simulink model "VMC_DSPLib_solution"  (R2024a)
settings: Solver=VariableStepDiscrete  StartTime=0.0  StopTime=5000  RelTol=1e-3
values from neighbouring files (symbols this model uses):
  cfi = NormalizeCoef(cf.Numerator,Kcf)    [CreateFilter.m]
  hb1 = NormalizeHBCoef(hb.Numerator,K1/2)    [CreateFilter.m]
  hb2 = NormalizeHBCoef(hb.Numerator,K2/2)    [CreateFilter.m]
  hb3 = NormalizeHBCoef(hb.Numerator,K3/2)    [CreateFilter.m]
  S = sum(round(C0))    [NormalizeCoef.m]
  Shift2 = 15    [CreateFilter.m]
  Shift3 = 15    [CreateFilter.m]
  ShiftCF = 15    [CreateFilter.m]
undefined symbols (not defined in the file or in its folder): aiecode_src, code, Evaluation, FreqShift, None, Platform, VCK190, Versal, vsva2197, xcvc1902
libraries: aieDSP x4, aieBasic x3, dspmlti4 x3, dspsrcs4 x1, aieUtilities x1, vmcUtilities x1

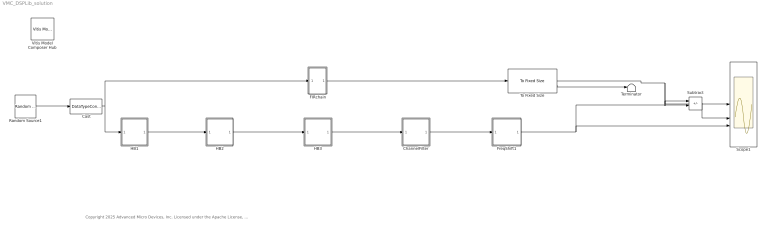
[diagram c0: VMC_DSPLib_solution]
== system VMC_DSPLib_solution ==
  note: Copyright 2025 Advanced Micro Devices, Inc. Licensed under the Apache License, Version 2.0 (the "License"); you may not use this file except in compliance with the License. You may obtain a copy of the License at http://www.apache.org/licenses/LICENSE-2.0 Unless required by applicable law or agreed to in writing, software distributed under the License is distributed on an "AS IS" BASIS, WITHOUT WARRANTIES OR CONDITIONS OF ANY KIND, either express or implied. See the License for the specific language governing permissions and limitations under the License.
  Cast : DataTypeConversion  OutDataTypeStr=int16
  ChannelFilter : Subsystem  mask{COEFFS=cfi, Shift=ShiftCF}
      mask prompts: COEFFS "Coefficients"; Shift "Final Shift"
  FIRchain : Subsystem
  FreqShift1 : Subsystem
  HB1 : Subsystem  mask{COEFFS=hb1, Shift=16}
      mask prompts: COEFFS "Coefficients"; Shift "Final Shift"
  HB2 : Subsystem  mask{COEFFS=hb2, Shift=Shift2}
      mask prompts: COEFFS "Coefficients"; Shift "Final Shift"
  HB3 : Subsystem  mask{COEFFS=hb3, Shift=Shift3}
      mask prompts: COEFFS "Coefficients"; Shift "Final Shift"
  Random Source1 : dspsrcs4/Random Source  SrcType=Uniform  MinVal=-30000  MaxVal=30000  MeanVal=0  VarVal=1  RepMode=Specify seed  rawSeed=1  IsInherit=off  SampTime=1  SampFrame=2048  OutComplex=Complex  DataType=double  SimulateUsing=Interpreted execution
  Scope1 : Scope  NumInputPorts=3
  Subtract : Sum  Inputs=+-
  Terminator : Terminator
  To Fixed Size : aieUtilities/To Fixed Size  Mode=Produce a valid output signal  OutputSize=256  CopyMethod=Buffer samples to form output  HasStatusOutput=on
  Vitis Model Composer Hub : vmcUtilities/Vitis Model Composer Hub  Tag=genX  CodeGeneration=off  SubsystemName=FIRchain  StartColumn=1  NumberOfColumns=1  TargetDirectory=./code  exportDesign=off  analyzeDesign=off  validateDesignOnHw=off  ExportType=AI Engines  IpVendor=xilinx.com  IpLibrary=hls  IpVersion=1.0  IpHWLanguage=Verilog  AieCompilerOptions={}  AieSimulatorOptions={}  CreateTestbench=on  TestbenchStackSize=10  RunRtlSim=off  RunCSim=off  RunAieSim=on  AieSimTimeout=50000  RunAieSimProfiling=on  LaunchVitisAnalyzer=on  PlotOutput=off  RunX86Sim=off  X86SimTimeout=10  GenHwImage=on  GenLibadfXo=off  GenHwValidationCode=off  PlatformType=Specify Platform  Platform=/opt/amd/Vitis/2024.2/base_platforms/xilinx_vck190_base_202420_1/xilinx_vck190_base_202420_1.xpfm  HwSystemType=Baremetal  HwValidationTarget=hw_emu  ProjDevice=Versal VCK190 Evaluation Platform (xcvc1902-vsva2197-2MP-e-S)  ProjDevicePart=xcvc1902-vsva2197-2MP-e-S  AIEType=AIE  SamplePeriod=-1  ClockFrequency=200  DataPathParallelism=1  xilinxfamily=versalaicore  part=xcvc1902  speed=-2MP-e-S  package=vsva2197  directory=./code  testbench=off  incr_netlist=off  synthesis_tool=Vivado  clock_wrapper=Clock Enables  dbl_ovrd=According to Block Masks  dcm_input_clock_period=10  sysclk_period=10  simulink_period=1  eval_field=0  IPInfoJsonString="{\"AIESubsystem\":{\"SubsystemName\":\"FIRchain\",\"TargetDirectory\":\"./code\",\"SubsystemDir\":\"./code/ip/FIRchain\"}}"  LogFileName=/home/amd/training/vmc_aie_dsplib/lab/VCK190/code/model_composer.log  NThreads=4
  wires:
  To Fixed Size/1 -> Subtract/1, Scope1/1
  Subtract/1 -> Scope1/2
  To Fixed Size/2 -> Terminator/1
  Cast/1 -> FIRchain/1(In1), HB1/1(In1)
  HB1/1(Out1) -> HB2/1(In1)
  HB2/1(Out1) -> HB3/1(In1)
  HB3/1(Out1) -> ChannelFilter/1(In1)
  ChannelFilter/1(Out1) -> FreqShift1/1(In1)
  FreqShift1/1(Out1) -> Subtract/2, Scope1/3
  FIRchain/1(Out1) -> To Fixed Size/1
  Random Source1/1 -> Cast/1

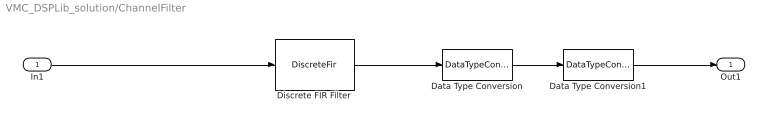
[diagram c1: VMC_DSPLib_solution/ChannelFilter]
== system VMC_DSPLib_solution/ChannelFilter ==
  In1 : Inport
  Data Type Conversion : DataTypeConversion  OutDataTypeStr=fixdt(1,32,Shift)  ConvertRealWorld=Stored Integer (SI)
  Data Type Conversion1 : DataTypeConversion  OutDataTypeStr=int16
  Discrete FIR Filter : DiscreteFir  Coefficients=COEFFS  InputProcessing=Columns as channels (frame based)
  Out1 : Outport
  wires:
  Data Type Conversion/1 -> Data Type Conversion1/1
  In1/1 -> Discrete FIR Filter/1
  Discrete FIR Filter/1 -> Data Type Conversion/1
  Data Type Conversion1/1 -> Out1/1

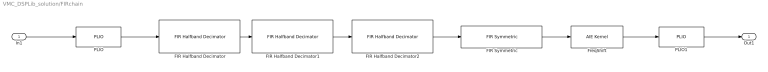
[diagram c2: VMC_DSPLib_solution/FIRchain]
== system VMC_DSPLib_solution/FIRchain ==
  In1 : Inport
  FIR Halfband Decimator : aieDSP/FIR Halfband Decimator  data_type=cint16  coef_type=int16  use_coeff_reload=off  dual_ip=off  num_outputs=off  coeff=hb1_aie  fir_length=31  input_window_size=2048  shift_val=16  rnd_mode=Floor  sat_mode=0-None  deci_poly=1  casc_length=2  AIE_VARIANT=1  blockJsonConstraints=[]  blockJsonConstraintsInternal=[]  spec=vmc_fir_decimate_hb.json  SerializedMaskParamNames=[]  SerializedMaskParamValues=[]  SerializedMaskParamVisibilities=[]  block_type=FIR Halfband Decimator  SerializedMaskParamDataypes=typename|typename|bool|bool|bool|coef_type|uint|uint|uint|uint|uint|uint|uint|uint  SerializedMaskParamEnumStrArr=0|0|0|0|0|0|0|0|0|Floor,Ceiling,Round to positive infinity,Round to negative infinity,Round symmetrical to infinity,Round symmetrical to zero,Round convergent to even,Round convergent to odd|0-None,1-Asymmetric,3-Symmetric|0|0|0  SerializedMaskParamEnumValArr=0|0|0|0|0|0|0|0|0|0,1,2,3,4,5,6,7|0,1,3|0|0|0  SerializedMaskParamVectorArr=0|0|0|0|0|1|0|0|0|0|0|0|0|0
  FIR Halfband Decimator1 : aieDSP/FIR Halfband Decimator  data_type=cint16  coef_type=int16  use_coeff_reload=off  dual_ip=off  num_outputs=off  coeff=hb2_aie  fir_length=31  input_window_size=1024  shift_val=Shift2  rnd_mode=Floor  sat_mode=0-None  deci_poly=1  casc_length=2  AIE_VARIANT=1  blockJsonConstraints=[]  blockJsonConstraintsInternal=[]  spec=vmc_fir_decimate_hb.json  SerializedMaskParamNames=[]  SerializedMaskParamValues=[]  SerializedMaskParamVisibilities=[]  block_type=FIR Halfband Decimator  SerializedMaskParamDataypes=typename|typename|bool|bool|bool|coef_type|uint|uint|uint|uint|uint|uint|uint|uint  SerializedMaskParamEnumStrArr=0|0|0|0|0|0|0|0|0|Floor,Ceiling,Round to positive infinity,Round to negative infinity,Round symmetrical to infinity,Round symmetrical to zero,Round convergent to even,Round convergent to odd|0-None,1-Asymmetric,3-Symmetric|0|0|0  SerializedMaskParamEnumValArr=0|0|0|0|0|0|0|0|0|0,1,2,3,4,5,6,7|0,1,3|0|0|0  SerializedMaskParamVectorArr=0|0|0|0|0|1|0|0|0|0|0|0|0|0
  FIR Halfband Decimator2 : aieDSP/FIR Halfband Decimator  data_type=cint16  coef_type=int16  use_coeff_reload=off  dual_ip=off  num_outputs=off  coeff=hb3_aie  fir_length=31  input_window_size=512  shift_val=Shift3  rnd_mode=Floor  sat_mode=0-None  deci_poly=1  casc_length=2  AIE_VARIANT=1  blockJsonConstraints=[]  blockJsonConstraintsInternal=[]  spec=vmc_fir_decimate_hb.json  SerializedMaskParamNames=[]  SerializedMaskParamValues=[]  SerializedMaskParamVisibilities=[]  block_type=FIR Halfband Decimator  SerializedMaskParamDataypes=typename|typename|bool|bool|bool|coef_type|uint|uint|uint|uint|uint|uint|uint|uint  SerializedMaskParamEnumStrArr=0|0|0|0|0|0|0|0|0|Floor,Ceiling,Round to positive infinity,Round to negative infinity,Round symmetrical to infinity,Round symmetrical to zero,Round convergent to even,Round convergent to odd|0-None,1-Asymmetric,3-Symmetric|0|0|0  SerializedMaskParamEnumValArr=0|0|0|0|0|0|0|0|0|0,1,2,3,4,5,6,7|0,1,3|0|0|0  SerializedMaskParamVectorArr=0|0|0|0|0|1|0|0|0|0|0|0|0|0
  FIR Symmetric : aieDSP/FIR Symmetric  data_type=cint16  coef_type=int16  use_coeff_reload=off  dual_ip=off  num_outputs=off  coeff=cfi_aie  fir_length=length(cfi)  input_window_size=256  shift_val=ShiftCF  rnd_mode=Floor  sat_mode=0-None  casc_length=1  AIE_VARIANT=1  blockJsonConstraints=[]  blockJsonConstraintsInternal=[]  spec=vmc_fir_sr_sym.json  SerializedMaskParamNames=[]  SerializedMaskParamValues=[]  SerializedMaskParamVisibilities=[]  block_type=FIR Symmetric  SerializedMaskParamDataypes=typename|typename|bool|bool|bool|coef_type|uint|uint|uint|uint|uint|uint|uint  SerializedMaskParamEnumStrArr=0|0|0|0|0|0|0|0|0|Floor,Ceiling,Round to positive infinity,Round to negative infinity,Round symmetrical to infinity,Round symmetrical to zero,Round convergent to even,Round convergent to odd|0-None,1-Asymmetric,3-Symmetric|0|0  SerializedMaskParamEnumValArr=0|0|0|0|0|0|0|0|0|0,1,2,3,4,5,6,7|0,1,3|0|0  SerializedMaskParamVectorArr=0|0|0|0|0|1|0|0|0|0|0|0|0
  FreqShift : aieBasic/AIE Kernel  KernelAllAttrs=s[12;12;9;9;19;14;21;23;21;23;24;21;15;17;12;24;26;26;26;27;28;9;21;23;23;23;24;25;14;19;19;29]@FunctionNameDeclFileNamePortNamesPortTypesPortSerializedTypesPortDirectionsPortWindowSizeEnablesPortWindowMarginEnablesPortBufferSizeEnablesPortBufferMarginEnablesPortSynchronicityEnablesPortSignalSizeEnablesPortBufferSizesPortBufferMarginsFunctionDeclFunctionTemplateSpecKindFunctionTemplateParamNamesFu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  PortNames={'in'; 'out'}  PortSerializedTypes={'{Q2{R{Tadf::input_buffer{1{t{Scint16}}}}}}'; '{Q2{R{Tadf::output_buffer{1{t{Scint16}}}}}}'}  PortWindowSizes={2.560000000000000000e+02, 2.560000000000000000e+02}  PortWindowMargins={0.000000000000000000e+00, 0.000000000000000000e+00}  PortSynchronicities={'sync', 'sync'}  PortSignalSizes={0.000000000000000000e+00; 0.000000000000000000e+00}  FunctionTemplateSpecKind=implicit  FunctionTemplateParamNames={'FRAME_LENGTH'}  FunctionTemplateParamKinds={'nontype'}  FunctionTemplateParamTypes={'int'}  FunctionTemplateParamValues={'256'}  FunctionIndex=1  FunctionTabVisible=on  FunctionTemplateParamsVisible=on  FunctionDeclTypeOptions=|  FunctionDecl=|  FunctionTemplateParams={ 'FRAME_LENGTH', 'int', '256' }  FunctionTemplateParamsEnables={'off', 'off', 'on'}  PortAttrs={ 'input', 'in', 'adf::input_buffer< cint16 > & restrict', '256', '0', 'sync', ''; 'output', 'out', 'adf::output_buffer< cint16 > & restrict', '256', '', 'sync', '' }  PortAttrsEnables={'off', 'off', 'off', 'on', 'off', 'off', 'off';'off', 'off', 'off', 'on', 'off', 'off', 'off'}  SampleTime=-1  KernelHeaderFile=aiecode_src/FreqShift.h  KernelFunction=FreqShift  KernelSourceFile=aiecode_src/FreqShift.cpp  KernelSearchPaths={}  PreProcOptions={}  blockJsonConstraints=[]
      | C[1 1]@t135@template < int FRAME_LENGTH > 
      | void FreqShift(adf::input_buffer< cint16 > && restrict in, adf::output_buffer< cint16 > && restrict out)
      | template < int FRAME_LENGTH > 
      | void FreqShift(adf::input_buffer< cint16 > && restrict in, adf::output_buffer< cint16 > && restrict out)
  PLIO : aieBasic/PLIO  PlioWidth=128  PlioFreqSpec=on  PlioFreq=250  ColLocation=0  channel=0  blockJsonConstraints=[]  deprecateConstraints=0
  PLIO1 : aieBasic/PLIO  PlioWidth=128  PlioFreqSpec=on  PlioFreq=250  ColLocation=0  channel=0  blockJsonConstraints=[]  deprecateConstraints=0
  Out1 : Outport
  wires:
  FIR Symmetric/1 -> FreqShift/1
  FIR Halfband Decimator2/1 -> FIR Symmetric/1
  FIR Halfband Decimator1/1 -> FIR Halfband Decimator2/1
  FIR Halfband Decimator/1 -> FIR Halfband Decimator1/1
  In1/1 -> PLIO/1
  PLIO/1 -> FIR Halfband Decimator/1
  FreqShift/1 -> PLIO1/1
  PLIO1/1 -> Out1/1

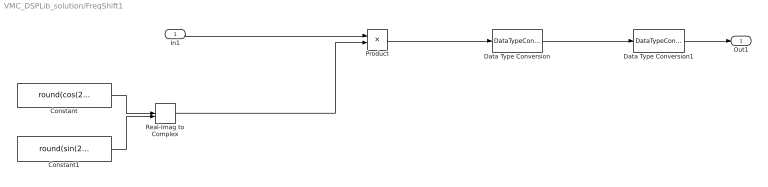
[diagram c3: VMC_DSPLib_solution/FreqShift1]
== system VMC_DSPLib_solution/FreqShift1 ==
  In1 : Inport
  Constant : Constant  Value=round(cos(2*pi*[0:255]/8)*16384)  SampleTime=2048
  Constant1 : Constant  Value=round(sin(2*pi*[0:255]/8)*16384)  SampleTime=2048
  Data Type Conversion : DataTypeConversion  OutDataTypeStr=fixdt(1,32,14)  ConvertRealWorld=Stored Integer (SI)
  Data Type Conversion1 : DataTypeConversion  OutDataTypeStr=int16
  Product : Product
  Real-Imag to Complex : RealImagToComplex
  Out1 : Outport
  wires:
  In1/1 -> Product/1
  Product/1 -> Data Type Conversion/1
  Real-Imag to Complex/1 -> Product/2
  Data Type Conversion1/1 -> Out1/1
  Constant/1 -> Real-Imag to Complex/1
  Constant1/1 -> Real-Imag to Complex/2
  Data Type Conversion/1 -> Data Type Conversion1/1

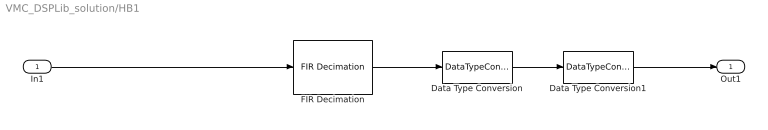
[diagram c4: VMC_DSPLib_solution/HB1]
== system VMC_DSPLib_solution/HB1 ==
  In1 : Inport
  Data Type Conversion : DataTypeConversion  OutDataTypeStr=fixdt(1,32,Shift)  ConvertRealWorld=Stored Integer (SI)
  Data Type Conversion1 : DataTypeConversion  OutDataTypeStr=int16
  FIR Decimation : dspmlti4/FIR Decimation  FilterSource=Dialog parameters  h=COEFFS  D=2  filtStruct=Direct form  FilterObject=FDECIM  InputProcessing=Columns as channels (frame based)  framing=Enforce single-rate processing  AllowArbitraryInputLength=off  inputOffset=0  outputBufInitCond=0  roundingMode=Floor  overflowMode=off  firstCoeffDataTypeStr=Inherit: Same word length as input  firstCoeffMin=[]  firstCoeffMax=[]  firstCoeffLastDataTypeStr=Inherit: Same word length as input  outputDataTypeStr=Inherit: Same as accumulator  outputMin=[]  outputMax=[]  outputLastDataTypeStr=Inherit: Same as accumulator
  Out1 : Outport
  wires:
  Data Type Conversion1/1 -> Out1/1
  FIR Decimation/1 -> Data Type Conversion/1
  In1/1 -> FIR Decimation/1
  Data Type Conversion/1 -> Data Type Conversion1/1

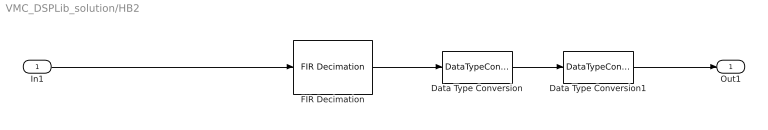
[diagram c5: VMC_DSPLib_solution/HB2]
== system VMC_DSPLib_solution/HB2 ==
  In1 : Inport
  Data Type Conversion : DataTypeConversion  OutDataTypeStr=fixdt(1,32,Shift)  ConvertRealWorld=Stored Integer (SI)
  Data Type Conversion1 : DataTypeConversion  OutDataTypeStr=int16
  FIR Decimation : dspmlti4/FIR Decimation  FilterSource=Dialog parameters  h=COEFFS  D=2  filtStruct=Direct form  FilterObject=FDECIM  InputProcessing=Columns as channels (frame based)  framing=Enforce single-rate processing  AllowArbitraryInputLength=off  inputOffset=0  outputBufInitCond=0  roundingMode=Floor  overflowMode=off  firstCoeffDataTypeStr=Inherit: Same word length as input  firstCoeffMin=[]  firstCoeffMax=[]  firstCoeffLastDataTypeStr=Inherit: Same word length as input  outputDataTypeStr=Inherit: Same as accumulator  outputMin=[]  outputMax=[]  outputLastDataTypeStr=Inherit: Same as accumulator
  Out1 : Outport
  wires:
  Data Type Conversion/1 -> Data Type Conversion1/1
  In1/1 -> FIR Decimation/1
  FIR Decimation/1 -> Data Type Conversion/1
  Data Type Conversion1/1 -> Out1/1

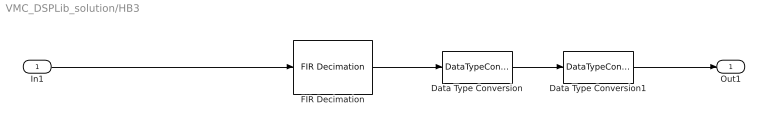
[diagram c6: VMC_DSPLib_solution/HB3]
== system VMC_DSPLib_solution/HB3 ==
  In1 : Inport
  Data Type Conversion : DataTypeConversion  OutDataTypeStr=fixdt(1,32,Shift)  ConvertRealWorld=Stored Integer (SI)
  Data Type Conversion1 : DataTypeConversion  OutDataTypeStr=int16
  FIR Decimation : dspmlti4/FIR Decimation  FilterSource=Dialog parameters  h=COEFFS  D=2  filtStruct=Direct form  FilterObject=FDECIM  InputProcessing=Columns as channels (frame based)  framing=Enforce single-rate processing  AllowArbitraryInputLength=off  inputOffset=0  outputBufInitCond=0  roundingMode=Floor  overflowMode=off  firstCoeffDataTypeStr=Inherit: Same word length as input  firstCoeffMin=[]  firstCoeffMax=[]  firstCoeffLastDataTypeStr=Inherit: Same word length as input  outputDataTypeStr=Inherit: Same as accumulator  outputMin=[]  outputMax=[]  outputLastDataTypeStr=Inherit: Same as accumulator
  Out1 : Outport
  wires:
  Data Type Conversion1/1 -> Out1/1
  FIR Decimation/1 -> Data Type Conversion/1
  In1/1 -> FIR Decimation/1
  Data Type Conversion/1 -> Data Type Conversion1/1
